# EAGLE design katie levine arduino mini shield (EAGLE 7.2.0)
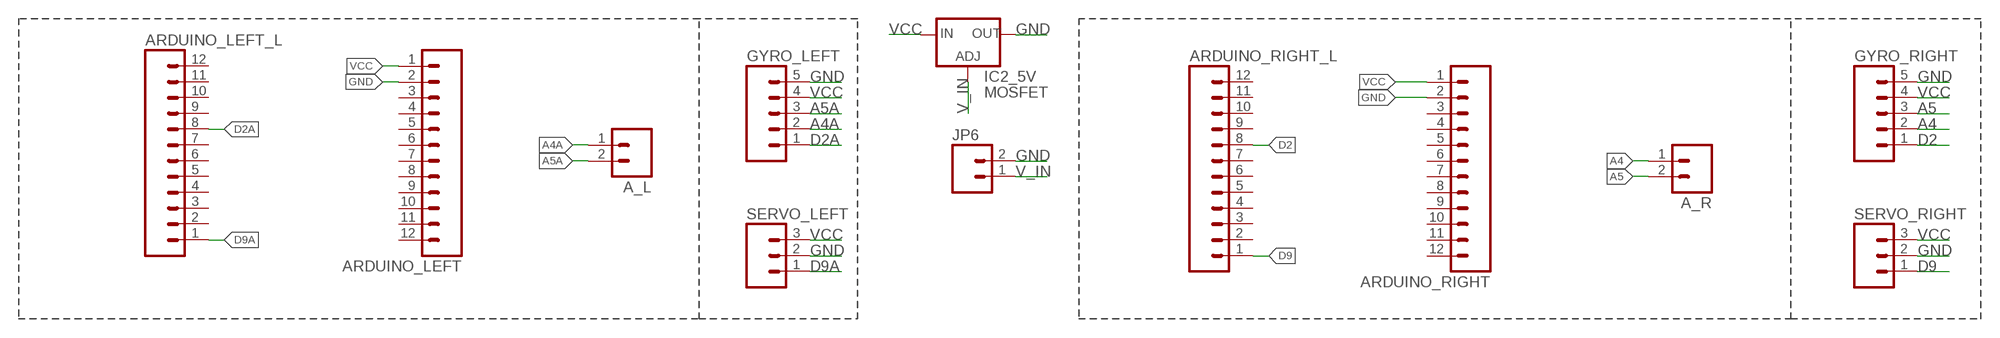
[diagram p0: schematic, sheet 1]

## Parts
A_L  M02PTH  [1X02]
A_R  M02PTH  [1X02]
ARDUINO_LEFT  M12PTH  [1X12]
ARDUINO_LEFT_L  M12PTH  [1X12]
ARDUINO_RIGHT  M12PTH  [1X12]
ARDUINO_RIGHT_L  M12PTH  [1X12]
GYRO_LEFT  M05LOCK  [1X05_LOCK]
GYRO_RIGHT  M05LOCK  [1X05_LOCK]
IC2_5V  MOSFET  V_REG_317SMD  [SOT223]
JP6  M02  [1X02_LONGPADS]
SERVO_LEFT  M03LOCK  [1X03_LOCK]
SERVO_RIGHT  M03LOCK  [1X03_LOCK]

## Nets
A4: A_R.1 GYRO_RIGHT.2
A4A: A_L.1 GYRO_LEFT.2
A5: A_R.2 GYRO_RIGHT.3
A5A: A_L.2 GYRO_LEFT.3
D2: ARDUINO_RIGHT_L.8 GYRO_RIGHT.1
D2A: ARDUINO_LEFT_L.8 GYRO_LEFT.1
D9: ARDUINO_RIGHT_L.1 SERVO_RIGHT.1
D9A: ARDUINO_LEFT_L.1 SERVO_LEFT.1
GND [vcc]: ARDUINO_LEFT.2 ARDUINO_RIGHT.2 GYRO_LEFT.5 GYRO_RIGHT.5 IC2_5V.2(OUT) JP6.2 SERVO_LEFT.2 SERVO_RIGHT.2
V_IN: IC2_5V.1(ADJ) JP6.1
VCC: ARDUINO_LEFT.1 ARDUINO_RIGHT.1 GYRO_LEFT.4 GYRO_RIGHT.4 IC2_5V.3(IN) SERVO_LEFT.3 SERVO_RIGHT.3
Unconnected: ARDUINO_LEFT.3 ARDUINO_LEFT.4 ARDUINO_LEFT.5 ARDUINO_LEFT.6 ARDUINO_LEFT.7 ARDUINO_LEFT.8 ARDUINO_LEFT.9 ARDUINO_LEFT.10 ARDUINO_LEFT.11 ARDUINO_LEFT.12 ARDUINO_LEFT_L.2 ARDUINO_LEFT_L.3 ARDUINO_LEFT_L.4 ARDUINO_LEFT_L.5 ARDUINO_LEFT_L.6 ARDUINO_LEFT_L.7 ARDUINO_LEFT_L.9 ARDUINO_LEFT_L.10 ARDUINO_LEFT_L.11 ARDUINO_LEFT_L.12 ARDUINO_RIGHT.3 ARDUINO_RIGHT.4 ARDUINO_RIGHT.5 ARDUINO_RIGHT.6 ARDUINO_RIGHT.7 ARDUINO_RIGHT.8 ARDUINO_RIGHT.9 ARDUINO_RIGHT.10 ARDUINO_RIGHT.11 ARDUINO_RIGHT.12 ARDUINO_RIGHT_L.2 ARDUINO_RIGHT_L.3 ARDUINO_RIGHT_L.4 ARDUINO_RIGHT_L.5 ARDUINO_RIGHT_L.6 ARDUINO_RIGHT_L.7 ARDUINO_RIGHT_L.9 ARDUINO_RIGHT_L.10 ARDUINO_RIGHT_L.11 ARDUINO_RIGHT_L.12

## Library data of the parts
A_L A_R = SparkFun:M02: Header 2
ARDUINO_LEFT ARDUINO_LEFT_L ARDUINO_RIGHT ARDUINO_RIGHT_L = SparkFun:M12: Header 12 Standard 12-pin 0.1" header. Use with straight break away headers (SKU : PRT-00116), right angle break away headers (PRT-00553), swiss pins (PRT-00743), machine pins (PRT-00117), and female headers (PRT-00115).
GYRO_LEFT GYRO_RIGHT = 01_SparkFun:M05: Header 5 Standard 5-pin 0.1" header. Use with straight break away headers (SKU : PRT-00116), right angle break away headers (PRT-00553), swiss pins (PRT-00743), machine pins (PRT-00117), and female headers (PRT-00115). Molex polarized connector foot print use with SKU : PRT-08230 with associated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
IC2_5V = 01_SparkFun:V_REG_317: Voltage Regulator Standard LM317 adjustable voltage regulator. AOI (Adjust Output Input). Google 'LM317 Calculator' for easy to use app to get the two resistor values needed. 240/720 for 5V output. 240/390 for 3.3V output. Spark Fun Electronics SKU : COM-00527
JP6 = 01_SparkFun:M02: Header 2
SERVO_LEFT SERVO_RIGHT = 01_SparkFun:M03: Header 3 Standard 3-pin 0.1" header. Use with straight break away headers (SKU : PRT-00116), right angle break away headers (PRT-00553), swiss pins (PRT-00743), machine pins (PRT-00117), and female headers (PRT-00115). Molex polarized connector foot print use with SKU : PRT-08232 with associated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

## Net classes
0 default: width 0.203 mm
1 vcc: width 0.254 mm

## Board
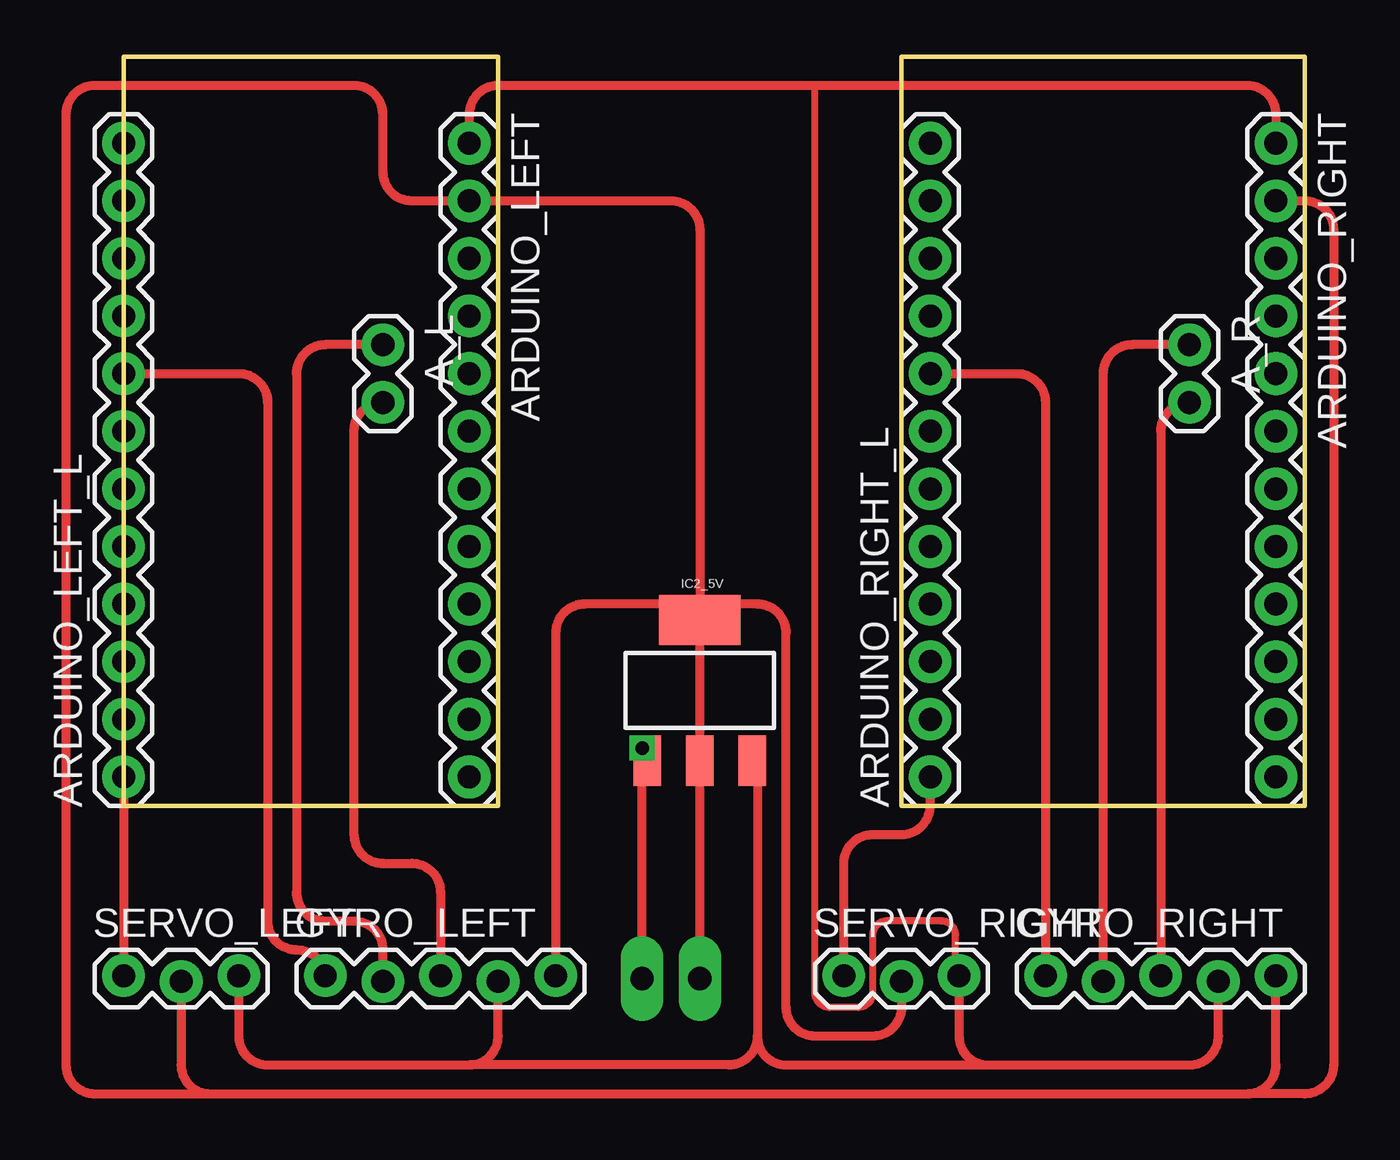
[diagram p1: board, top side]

Size 52.07 x 33.02 mm. Coordinates in mm from the lower left corner, seen from the top.
Outline: 16.51,33.02 0,33.02 0,0 16.51,0 16.51,33.02
Outline: 52.07,33.02 34.29,33.02 34.29,0 52.07,0 52.07,33.02
Copper layers (1*16): Top 0.035mm / dielectric 1.5mm / Bottom 0.035mm
Design rules "SparkFun-2-layer *": minimum track width 7mil, minimum drill 15mil, track to track 8mil, track to pad 8mil, pad to pad 8mil, via to via 8mil, smd to smd 8mil, copper to edge 8mil, drill to drill 8mil, minimum pad ring 12mil, minimum via ring 10mil, stop-mask expansion 4mil, vias tented up to drill 20mil, thermal gap 10mil

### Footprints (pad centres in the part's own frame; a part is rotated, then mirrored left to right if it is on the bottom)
1X02 = drill 1.016 pad 1.88: 1 0,0; 2 2.54,0
1X12 = drill 1.016 pad 1.88: 1 0,0; 2 2.54,0; 3 5.08,0; 4 7.62,0; 5 10.16,0; 6 12.7,0; 7 15.24,0; 8 17.78,0; 9 20.32,0; 10 22.86,0; 11 25.4,0; 12 27.94,0
1X05_LOCK = drill 1.016 pad 1.88: 1 0,0.127; 2 2.54,-0.127; 3 5.08,0.127; 4 7.62,-0.127; 5 10.16,0.127
SOT223 = smd 1.219 x 2.235: 1 -2.311,-3.099; 2 0,-3.099; 3 2.311,-3.099 | smd 3.6 x 2.2: 4 0,3.099
1X02_LONGPADS = drill 1.016 pad 1.88 long: 1 0,0; 2 2.54,0
1X03_LOCK = drill 1.016 pad 1.88: 1 0,0.127; 2 2.54,-0.127; 3 5.08,0.127

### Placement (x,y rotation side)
A_L  11.43,20.32 270 top
A_R  46.99,20.32 270 top
ARDUINO_LEFT  15.24,29.21 270 top
ARDUINO_LEFT_L  0,1.27 90 top
ARDUINO_RIGHT  50.8,29.21 270 top
ARDUINO_RIGHT_L  35.56,1.27 90 top
GYRO_LEFT  8.89,-7.62 0 top  (outside the outline)
GYRO_RIGHT  40.64,-7.62 0 top  (outside the outline)
IC2_5V  25.4,5.08 0 top
JP6  22.86,-7.62 0 top  (outside the outline)
SERVO_LEFT  0,-7.62 0 top  (outside the outline)
SERVO_RIGHT  31.75,-7.62 0 top  (outside the outline)

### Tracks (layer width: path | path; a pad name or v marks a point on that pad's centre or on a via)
A4
  Top 0.406: A_R.1 44.45,20.32 arc90 43.18,19.05 GYRO_RIGHT.2
A4A
  Top 0.406: A_L.1 8.89,20.32 arc90 7.62,19.05 7.62,-3.81 arc90 8.89,-5.08 10.16,-5.08 arc-90 11.43,-6.35 GYRO_LEFT.2
A5
  Top 0.406: A_R.2 arc90 45.72,16.51 GYRO_RIGHT.3
A5A
  Top 0.406: A_L.2 arc90 10.16,16.51 10.16,-1.27 arc90 11.43,-2.54 12.7,-2.54 arc-90 13.97,-3.81 GYRO_LEFT.3
D2
  Top 0.406: ARDUINO_RIGHT_L.8 39.37,19.05 arc-90 40.64,17.78 GYRO_RIGHT.1
D2A
  Top 0.406: ARDUINO_LEFT_L.8 5.08,19.05 arc-90 6.35,17.78 6.35,-5.08 arc90 7.62,-6.35 arc-84 GYRO_LEFT.1
D9
  Top 0.406: SERVO_RIGHT.1 31.75,-2.54 arc-90 33.02,-1.27 34.29,-1.27 arc90 35.56,0 ARDUINO_RIGHT_L.1
D9A
  Top 0.406: ARDUINO_LEFT_L.1 SERVO_LEFT.1
GND
  Top 0.406: JP6.2 IC2_5V.2 25.4,8.89 | SERVO_LEFT.2 2.54,-11.43 arc90 3.81,-12.7 | 3.81,-12.7 49.53,-12.7 | 49.53,-12.7 arc90 50.8,-11.43 GYRO_RIGHT.5 | 25.4,8.89 20.32,8.89 arc90 19.05,7.62 GYRO_LEFT.5 | ARDUINO_RIGHT.2 52.07,26.67 arc-90 53.34,25.4 53.34,-11.43 arc-90 52.07,-12.7 49.53,-12.7 | 25.4,8.89 25.4,25.4 arc90 24.13,26.67 ARDUINO_LEFT.2 12.7,26.67 arc-90 11.43,27.94 11.43,30.48 arc90 10.16,31.75 -1.27,31.75 arc90 -2.54,30.48 -2.54,-11.43 arc90 -1.27,-12.7 3.81,-12.7 | SERVO_RIGHT.2 34.29,-8.89 arc-90 33.02,-10.16 30.48,-10.16 arc-90 29.21,-8.89 29.21,7.62 arc90 27.94,8.89 25.4,8.89
V_IN  (via drill 0.6)
  Top 0.203: IC2_5V.1 23.06,2.03 22.96,2.03 v22.86,2.54
  Top 0.406: JP6.1 v22.86,2.54
VCC
  Top 0.203: 36.68,-7.42 SERVO_RIGHT.3
  Top 0.305: 36.68,-7.42 36.68,-5.71 arc90 36.04,-5.08 33.66,-5.08 arc90 33.02,-5.71 33.02,-8.25 arc-90 32.38,-8.89 31.12,-8.89 arc-90 30.48,-8.25 30.48,31.75
  Top 0.406: SERVO_LEFT.3 5.08,-10.16 arc90 6.35,-11.43 15.24,-11.43 | 15.24,-11.43 arc90 16.51,-10.16 GYRO_LEFT.4 | IC2_5V.3 arc-90 27.94,1.75 27.94,-10.16 | 27.94,-10.16 arc-90 26.67,-11.43 15.24,-11.43 | SERVO_RIGHT.3 36.83,-10.16 arc90 38.1,-11.43 | 38.1,-11.43 46.99,-11.43 arc90 48.26,-10.16 GYRO_RIGHT.4 | 27.94,-10.16 arc90 29.21,-11.43 38.1,-11.43 | ARDUINO_LEFT.1 15.24,30.48 arc-90 16.51,31.75 30.48,31.75 49.53,31.75 arc-90 50.8,30.48 ARDUINO_RIGHT.1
